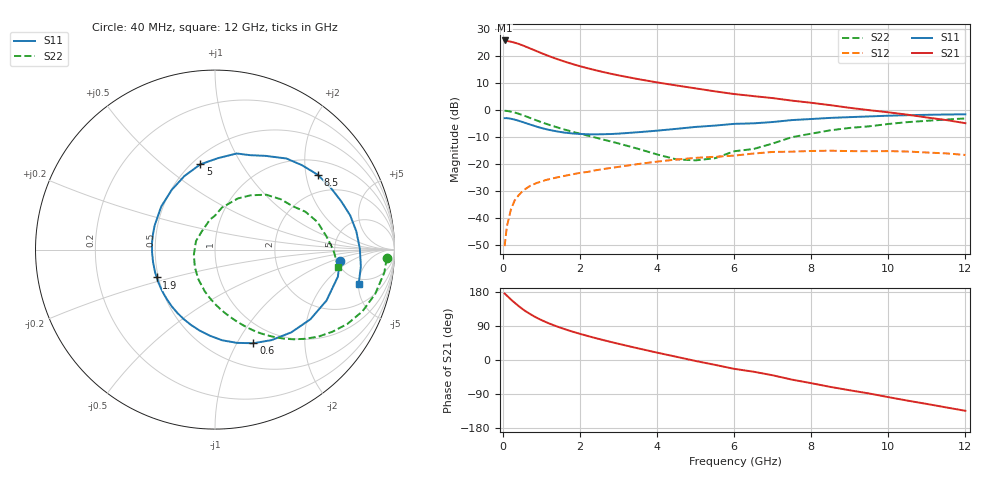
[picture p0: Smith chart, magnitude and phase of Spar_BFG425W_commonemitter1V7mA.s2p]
! Filename: 17bfg425.001
! BFG425W Field C1
! V1=8.436E-001V,V2=1.000E+000V, I1=1.005E-004A, I2=7.010E-003A
# GHz  S  MA  R 50
!  S11  S21  S12  S22
!Freq(GHz)  Mag  Ang  Mag  Ang  Mag  Ang  Mag  Ang
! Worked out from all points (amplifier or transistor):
!   44 points, 40 MHz to 12 GHz, reference 50 ohm
!   highest |S21| = 25.6 dB at 40 MHz (marker M1)
!   |S21| within 3 dB of that: start of sweep to 709 MHz
!   unconditionally stable (mu >= 1): 2.1 GHz to end of sweep
!   at 700 MHz: K = 0.44, MSG = 25.4 dB, |S12| = -28.2 dB
!   at 2.4 GHz: K = 1.07, MAG = 16.9 dB, |S12| = -22.4 dB
!   at 12 GHz: K = 1.43, MAG = 2.0 dB, |S12| = -16.7 dB
!   S11 on the Smith chart (normalised r, x): 40 MHz: 5.32, -1.29; 600 MHz: 0.77, -1.17; 1.9 GHz: 0.49, -0.17; 5 GHz: 0.55, +0.68; 8.5 GHz: 1.39, +2.33; 12 GHz: 4.21, -5.00
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0.04  0.699 -5.1  19.15 175.6  0.003 82.4  0.958 -2.9
0.2  0.683 -24.6  18.17 160.0  0.014 76.6  0.926 -15.5
0.3  0.658 -36.2  17.46 151.2  0.021 70.6  0.891 -22.6
0.4  0.627 -47.4  16.56 142.7  0.026 65.1  0.847 -29.2
0.5  0.595 -57.9  15.62 134.8  0.031 60.6  0.799 -34.9
0.6  0.564 -67.7  14.6 127.8  0.035 56.6  0.753 -40.1
0.8  0.507 -85.4  12.75 115.5  0.042 50.2  0.664 -48.8
0.9  0.481 -93.3  11.91 110.1  0.045 47.8  0.624 -52.6
1.1  0.44 -107.9  10.43 100.6  0.05 43.8  0.556 -59.0
1.3  0.41 -120.9  9.211 92.3  0.054 40.8  0.499 -64.6
1.5  0.387 -133.0  8.215 84.9  0.058 38.5  0.451 -69.4
1.9  0.36 -154.5  6.691 71.9  0.066 34.7  0.376 -78.4
2.2  0.352 -168.7  5.848 63.3  0.071 32.1  0.332 -85.0
3  0.362 158.5  4.328 42.7  0.088 24.5  0.238 -104.1
3.5  0.384 141.3  3.698 30.8  0.099 18.9  0.19 -119.1
4.5  0.444 112.5  2.818 8.5  0.12 6.0  0.121 -166.6
5  0.482 99.8  2.486 -2.6  0.129 -1.8  0.116 156.0
6.5  0.561 69.7  1.79 -30.9  0.155 -19.3  0.188 90.4
7.5  0.645 51.9  1.475 -51.8  0.168 -38.0  0.312 65.9
8.5  0.708 36.1  1.216 -71.1  0.175 -54.4  0.418 47.0
10.5  0.794 7.4  0.81 -107.2  0.169 -87.8  0.591 15.1
12  0.823 -13.5  0.565 -134.0  0.146 -116.3  0.692 -7.9
